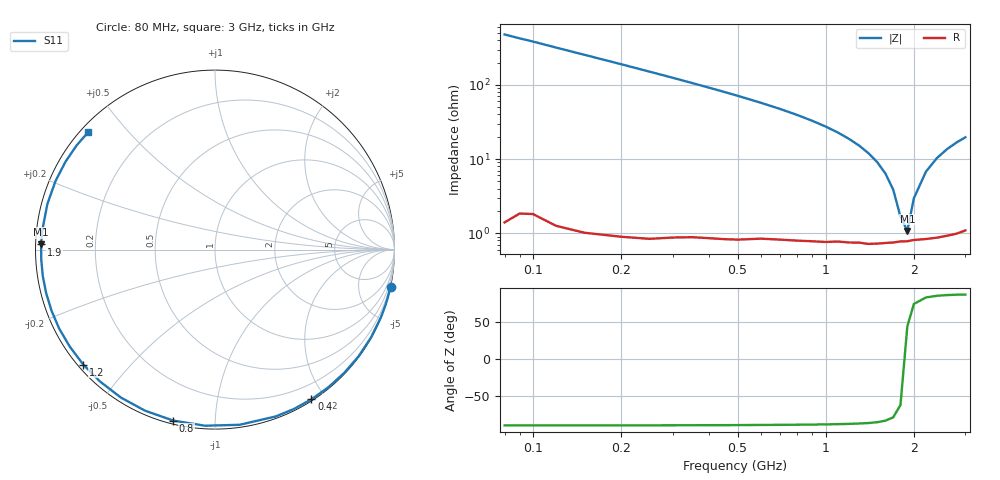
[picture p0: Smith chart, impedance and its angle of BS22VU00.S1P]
! SIEMENS Small Signal Semiconductors
! BB640
! Si Tuning Diode in SOD323
! VR = 22 V
! S-Parameters:  July  1993
# GHz  S  MA  R  50
!  f  S11
! GHz  MAG  ANG
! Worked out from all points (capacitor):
!   33 points, 80 MHz to 3 GHz, reference 50 ohm
!   read as one part to ground: C = 4.14 pF near 80 MHz
!   lowest |Z| = 1.07 ohm at 1.9 GHz (marker M1)
!   series resonance near 1.867 GHz, so ESL is about 1.8 nH
!   S11 on the Smith chart (normalised r, x): 80 MHz: 0.03, -9.59; 400 MHz: 0.02, -1.83; 800 MHz: 0.02, -0.79; 1.2 GHz: 0.01, -0.37; 1.9 GHz: 0.02, +0.01; 3 GHz: 0.02, +0.39
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0.08  0.9994 -11.9
0.15  0.9985 -22.2
0.2  0.9977 -29.4
0.25  0.9967 -36.6
0.3  0.9952 -43.6
0.35  0.9936 -50.5
0.4  0.9922 -57.2
0.45  0.9908 -63.7
0.5  0.9893 -70.0
0.6  0.9856 -82.0
0.7  0.9829 -93.2
0.8  0.9806 -103.7
0.9  0.9785 -113.5
1  0.9769 -122.5
1.1  0.9748 -131.0
1.2  0.9741 -138.9
1.3  0.9731 -146.2
1.4  0.9733 -153.1
1.5  0.9724 -159.5
1.6  0.9714 -165.6
1.7  0.9707 -171.3
1.9  0.9694 178.3
2  0.9683 173.5
2.2  0.9678 164.7
2.4  0.9672 156.7
2.6  0.9662 149.5
2.8  0.9652 143.0
3  0.963 137.1
